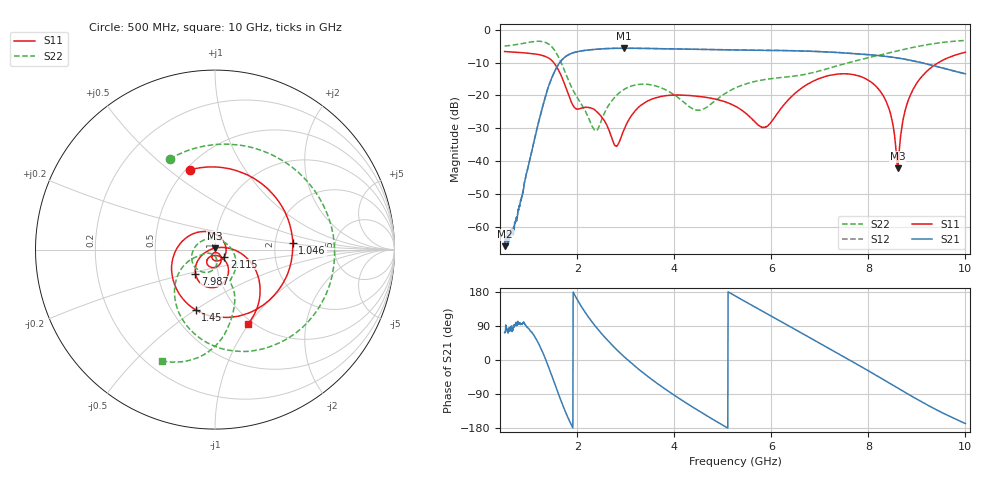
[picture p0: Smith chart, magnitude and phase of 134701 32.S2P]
!  2-Port S-parameters saved by WinCal
! VAR MeasName=S-Parameters (CALIBRATED_DATA) read from VNA (N5242A)
! VAR MeasDate=2013-7-3 16:33:23
! VAR NAME=134701 32
! VAR FILENAME=134701 32.S2P
! VAR DATE=2013-7-3 16:33:23
! VAR PHYS_PORTS=1,2
# Hz S MA R 50
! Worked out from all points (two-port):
!   1601 points, 500 MHz to 10 GHz, reference 50 ohm
!   highest |S21| = -5.63 dB at 2.952 GHz (marker M1); lowest = -65.9 dB at 511.9 MHz (marker M2)
!   |S21| within 3 dB of the highest: 1.72 GHz to 8.617 GHz (6.897 GHz wide, 133 % of centre)
!   lowest |S11| = -42.2 dB at 8.605 GHz (marker M3), VSWR 1.02, Z = 49.8 + j0.754 ohm
!   |S11| at or under -10 dB: 1.511 GHz to 9.447 GHz (7.936 GHz wide, 145 % of centre)
!   |S22| runs from -30.8 to -3.3 dB; largest |S21 - S12| = 0.0025
!   S11 on the Smith chart (normalised r, x): 500 MHz: 0.52, +0.59; 1.046 GHz: 2.52, +0.22; 1.45 GHz: 0.65, -0.50; 2.115 GHz: 1.10, -0.09; 7.987 GHz: 0.78, -0.21; 10 GHz: 0.94, -0.99
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5e8  0.4657 107.6  0.0005907 72.6  0.0006179 71.1  0.5644 116.6
5.11875e8  0.465 105.7  0.0005054 73.8  0.0007143 83.7  0.5657 114.9
7.196875e8  0.4545 70.8  0.001151 92.8  0.001143 91.0  0.5908 83.7
1.04625e9  0.435 4.8  0.01261 74.6  0.01265 74.7  0.6514 23.0
1.45e9  0.3524 -107.8  0.1681 -33.4  0.1682 -33.7  0.572 -80.2
1.71125e9  0.1672 154.1  0.3655 -123.3  0.3651 -123.3  0.263 -143.8
2.085312e9  0.06425 -26.6  0.477 140.5  0.4771 140.5  0.07261 -158.5
2.115e9  0.0647 -37.5  0.4806 134.5  0.4807 134.5  0.06707 -158.3
2.394062e9  0.05719 -100.1  0.5038 85.6  0.5042 85.5  0.02919 -111.0
2.785938e9  0.01709 -93.0  0.5213 30.3  0.5217 30.2  0.09628 -87.8
2.952188e9  0.02874 -48.9  0.5232 10.0  0.5226 10.0  0.122 -100.2
3.670625e9  0.09445 -81.6  0.5155 -64.0  0.5149 -64.0  0.1356 -163.8
4.49e9  0.09702 -112.9  0.5023 -133.2  0.5032 -133.2  0.05953 76.2
5.25e9  0.0687 -127.8  0.4923 169.4  0.4926 169.4  0.1294 -26.5
5.873438e9  0.03286 -83.8  0.4854 124.7  0.4857 124.6  0.1748 -55.0
6.835312e9  0.1612 -63.8  0.4696 55.7  0.4701 55.7  0.2205 -64.9
7.987188e9  0.1726 -129.1  0.4188 -27.5  0.4185 -27.8  0.3728 -74.8
8.420625e9  0.06429 -161.4  0.3885 -60.0  0.3872 -60.2  0.443 -80.9
8.604688e9  0.007718 101.4  0.3717 -73.9  0.3712 -74.0  0.4777 -83.8
8.765e9  0.06194 10.0  0.3544 -86.0  0.3542 -86.1  0.508 -86.8
8.996562e9  0.1533 -9.4  0.3273 -103.1  0.3264 -103.2  0.5532 -91.6
1e10  0.4541 -66.4  0.2132 -167.5  0.2131 -167.7  0.6867 -115.6
